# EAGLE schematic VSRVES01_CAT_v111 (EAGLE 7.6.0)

## Sheet 1 of 4: VSRV+DDR2
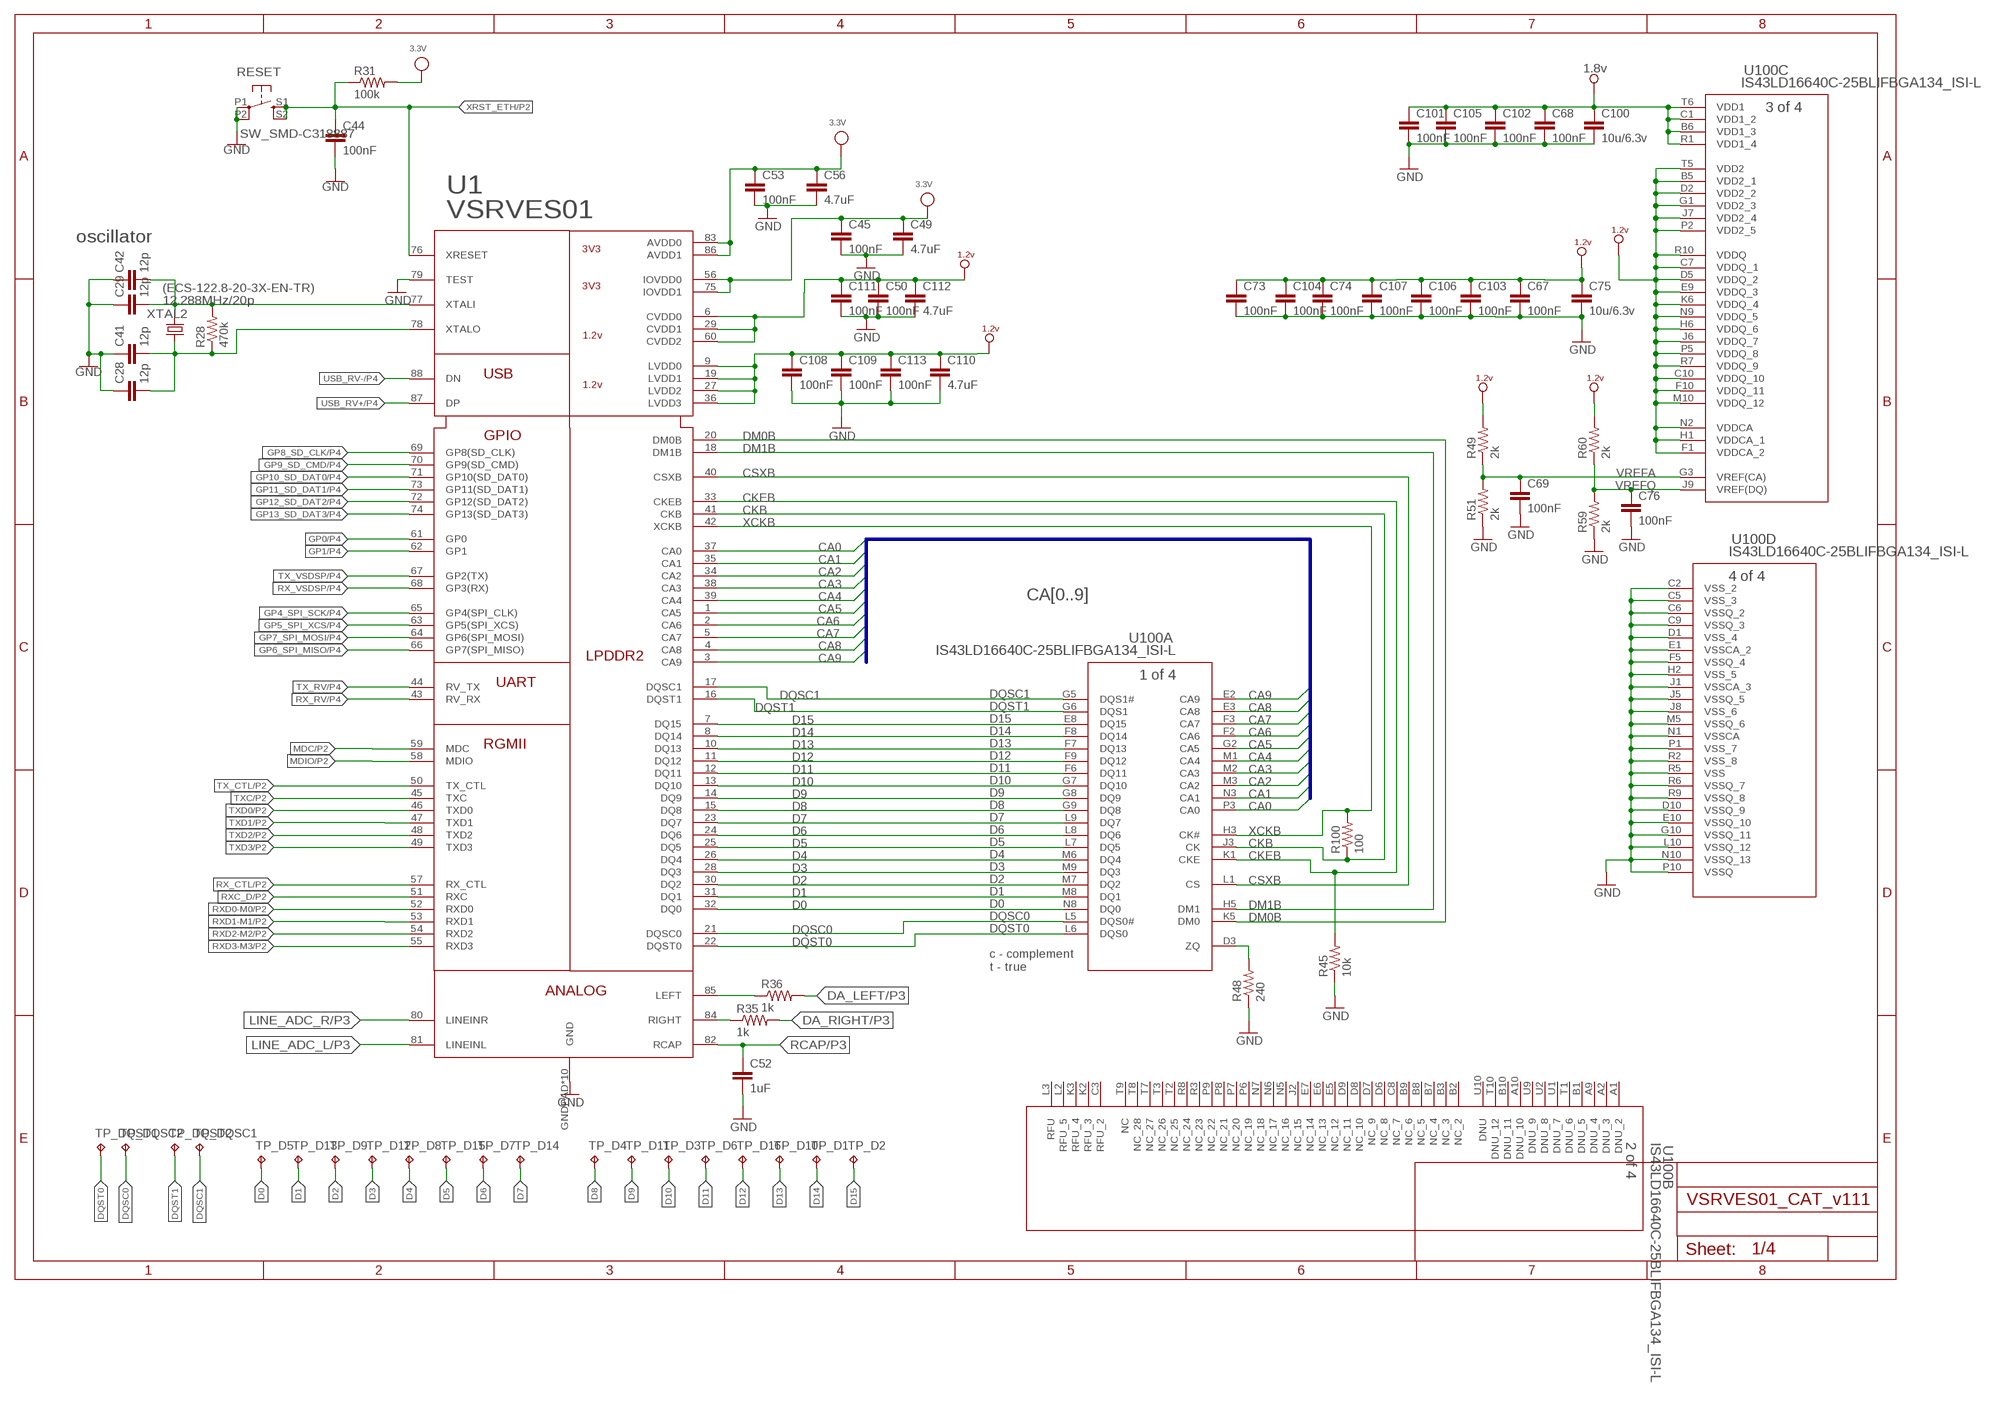
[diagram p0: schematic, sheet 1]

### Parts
C28  12p  C-EUC0603K  [C0603K]
C29  12p  C-EUC0603K  [C0603K]
C41  12p  C-EUC0603K  [C0603K]
C42  12p  C-EUC0603K  [C0603K]
C44  100nF  C-EUC0603K  [C0603K]
C45  100nF  C-EUC0603K  [C0603K]
C49  4.7uF  C-EUC0603K  [C0603K]
C50  100nF  C-EUC0603K  [C0603K]
C52  1uF  C-EUC0603K  [C0603K]
C53  100nF  C-EUC0603K  [C0603K]
C56  4.7uF  C-EUC0603K  [C0603K]
C67  100nF  C-EUC0603K  [C0603K]
C68  100nF  C-EUC0603K  [C0603K]
C69  100nF  C-EUC0603K  [C0603K]
C73  100nF  C-EUC0603K  [C0603K]
C74  100nF  C-EUC0603K  [C0603K]
C75  10u/6.3v  C-EUC0603K  [C0603K]
C76  100nF  C-EUC0603K  [C0603K]
C100  10u/6.3v  C-EUC0603K  [C0603K]
C101  100nF  C-EUC0603K  [C0603K]
C102  100nF  C-EUC0603K  [C0603K]
C103  100nF  C-EUC0603K  [C0603K]
C104  100nF  C-EUC0603K  [C0603K]
C105  100nF  C-EUC0603K  [C0603K]
C106  100nF  C-EUC0603K  [C0603K]
C107  100nF  C-EUC0603K  [C0603K]
C108  100nF  C-EUC0603K  [C0603K]
C109  100nF  C-EUC0603K  [C0603K]
C110  4.7uF  C-EUC0603K  [C0603K]
C111  100nF  C-EUC0603K  [C0603K]
C112  4.7uF  C-EUC0603K  [C0603K]
C113  100nF  C-EUC0603K  [C0603K]
R28  470k  R-US_R0603  [R0603]
R31  100k  R-US_R0603  [R0603]
R35  1k  R-US_R0603  [R0603]
R36  1k  R-US_R0603  [R0603]
R45  10k  R-US_R0603  [R0603]
R48  240  R-US_R0603  [R0603]
R49  2k  R-US_R0603  [R0603]
R51  2k  R-US_R0603  [R0603]
R59  2k  R-US_R0603  [R0603]
R60  2k  R-US_R0603  [R0603]
R100  100  R-US_R0603  [R0603]
RESET  SW_SMD-C318887  SW_SMD-SW-4_5.1X5.1X2.5_TS-1187A-C-E-B  [SW_SMD-SW-4_5.1X5.1X2.5_TS-1187A-C-E-B]
TP_D1  TPTP10R  [TP10R]
TP_D2  TPTP10R  [TP10R]
TP_D3  TPTP06R  [TP06R]
TP_D4  TPTP06R  [TP06R]
TP_D5  TPTP10R  [TP10R]
TP_D6  TPTP06R  [TP06R]
TP_D7  TPTP10R  [TP10R]
TP_D8  TPTP10R  [TP10R]
TP_D9  TPTP10R  [TP10R]
TP_D10  TPTP10R  [TP10R]
TP_D11  TPTP06R  [TP06R]
TP_D12  TPTP10R  [TP10R]
TP_D13  TPTP10R  [TP10R]
TP_D14  TPTP06R  [TP06R]
TP_D15  TPTP10R  [TP10R]
TP_D16  TPTP10R  [TP10R]
TP_DQSC1  TPTP06R  [TP06R]
TP_DQSC2  TPTP06R  [TP06R]
TP_DQST1  TPTP06R  [TP06R]
TP_DQST2  TPTP06R  [TP06R]
U1  VSRVES01  [QFN88_NEW2Q]
U100  IS43LD16640C-25BLIFBGA134_ISI-L  [FBGA134_ISI-L]
XTAL2  12.288MHz/20p  CRYSTAL  [CSM-3X]

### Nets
1.2V: C50.1 C67.1 C73.1 C74.1 C75.1 C103.1 C104.1 C106.1 C107.1 C108.1 C109.1 C110.1 C111.1 C112.1 C113.1 R49.2 R60.2 U1.6(CVDD0) U1.9(LVDD0) U1.19(LVDD1) U1.27(LVDD2) U1.29(CVDD1) U1.36(LVDD3) U1.60(CVDD2) U100.B5(C:VDD2_1) U100.C7(C:VDDQ_1) U100.C10(C:VDDQ_10) U100.D2(C:VDD2_2) U100.D5(C:VDDQ_2) U100.E9(C:VDDQ_3) U100.F1(C:VDDCA_2) U100.F10(C:VDDQ_11) U100.G1(C:VDD2_3) U100.H1(C:VDDCA_1) U100.H6(C:VDDQ_6) U100.J6(C:VDDQ_7) U100.J7(C:VDD2_4) U100.K6(C:VDDQ_4) U100.M10(C:VDDQ_12) U100.N2(C:VDDCA) U100.N9(C:VDDQ_5) U100.P2(C:VDD2_5) U100.P5(C:VDDQ_8) U100.R7(C:VDDQ_9) U100.R10(C:VDDQ) U100.T5(C:VDD2) ; supply symbol labelled +1.2V ; also sheet 2,4
1.8V: C68.1 C100.1 C101.1 C102.1 C105.1 U100.B6(C:VDD1_3) U100.C1(C:VDD1_2) U100.R1(C:VDD1_4) U100.T6(C:VDD1) ; supply symbol labelled +1.8V ; also sheet 4
3.3V: C45.1 C49.1 C53.1 C56.1 R31.2 U1.56(IOVDD0) U1.75(IOVDD1) U1.83(AVDD0) U1.86(AVDD1) ; also sheet 2,3,4
CA0: U1.37(CA0) U100.P3(A:CA0)
CA1: U1.35(CA1) U100.N3(A:CA1)
CA2: U1.34(CA2) U100.M3(A:CA2)
CA3: U1.38(CA3) U100.M2(A:CA3)
CA4: U1.39(CA4) U100.M1(A:CA4)
CA5: U1.1(CA5) U100.G2(A:CA5)
CA6: U1.2(CA6) U100.F2(A:CA6)
CA7: U1.5(CA7) U100.F3(A:CA7)
CA8: U1.4(CA8) U100.E3(A:CA8)
CA9: U1.3(CA9) U100.E2(A:CA9)
CKB: R100.1 U1.41(CKB) U100.J3(A:CK)
CKEB: R45.2 U1.33(CKEB) U100.K1(A:CKE)
CSXB: U1.40(CSXB) U100.L1(A:CS)
D0: TP_D5.TP U1.32(DQ0) U100.N8(A:DQ0)
D1: TP_D13.TP U1.31(DQ1) U100.M8(A:DQ1)
D2: TP_D9.TP U1.30(DQ2) U100.M7(A:DQ2)
D3: TP_D12.TP U1.28(DQ3) U100.M9(A:DQ3)
D4: TP_D8.TP U1.26(DQ4) U100.M6(A:DQ4)
D5: TP_D15.TP U1.25(DQ5) U100.L7(A:DQ5)
D6: TP_D7.TP U1.24(DQ6) U100.L8(A:DQ6)
D7: TP_D14.TP U1.23(DQ7) U100.L9(A:DQ7)
D8: TP_D4.TP U1.15(DQ8) U100.G9(A:DQ8)
D9: TP_D11.TP U1.14(DQ9) U100.G8(A:DQ9)
D10: TP_D3.TP U1.13(DQ10) U100.G7(A:DQ10)
D11: TP_D6.TP U1.12(DQ11) U100.F6(A:DQ11)
D12: TP_D16.TP U1.11(DQ12) U100.F9(A:DQ12)
D13: TP_D10.TP U1.10(DQ13) U100.F7(A:DQ13)
D14: TP_D1.TP U1.8(DQ14) U100.F8(A:DQ14)
D15: TP_D2.TP U1.7(DQ15) U100.E8(A:DQ15)
DA_LEFT: R36.2 ; also sheet 3
DA_RIGHT: R35.2 ; also sheet 3
DM0B: U1.20(DM0B) U100.K5(A:DM0)
DM1B: U1.18(DM1B) U100.H5(A:DM1)
DQSC0: TP_DQSC2.TP U1.21(DQSC0) U100.L5(A:DQS0#)
DQSC1: TP_DQSC1.TP U1.17(DQSC1) U100.G5(A:DQS1#)
DQST0: TP_DQST1.TP U1.22(DQST0) U100.L6(A:DQS0)
DQST1: TP_DQST2.TP U1.16(DQST1) U100.G6(A:DQS1)
GND: C28.1 C29.1 C41.1 C42.1 C44.2 C45.2 C49.2 C50.2 C52.2 C53.2 C56.2 C67.2 C68.2 C69.2 C73.2 C74.2 C75.2 C76.2 C100.2 C101.2 C102.2 C103.2 C104.2 C105.2 C106.2 C107.2 C108.2 C109.2 C110.2 C111.2 C112.2 C113.2 R45.1 R48.1 R51.1 R59.1 RESET.P1 RESET.P2 U1.79(TEST) U1.GNDPAD(GND) U1.P$1(GND) U1.P$2(GND) U1.P$3(GND) U1.P$4(GND) U1.P$5(GND) U1.P$6(GND) U1.P$7(GND) U1.P$8(GND) U1.P$9(GND) U100.C2(D:VSS_2) U100.C5(D:VSS_3) U100.C6(D:VSSQ_2) U100.C9(D:VSSQ_3) U100.D1(D:VSS_4) U100.D10(D:VSSQ_9) U100.E1(D:VSSCA_2) U100.E10(D:VSSQ_10) U100.F5(D:VSSQ_4) U100.G10(D:VSSQ_11) U100.H2(D:VSS_5) U100.J1(D:VSSCA_3) U100.J5(D:VSSQ_5) U100.J8(D:VSS_6) U100.L10(D:VSSQ_12) U100.M5(D:VSSQ_6) U100.N1(D:VSSCA) U100.N10(D:VSSQ_13) U100.P1(D:VSS_7) U100.P10(D:VSSQ) U100.R2(D:VSS_8) U100.R5(D:VSS) U100.R6(D:VSSQ_7) U100.R9(D:VSSQ_8) ; also sheet 2,3,4
GP0: U1.61(GP0) ; also sheet 4
GP1: U1.62(GP1) ; also sheet 4
GP4_SPI_SCK: U1.65(GP4(SPI_CLK)) ; also sheet 4
GP5_SPI_XCS: U1.63(GP5(SPI_XCS)) ; also sheet 4
GP6_SPI_MISO: U1.66(GP7(SPI_MISO)) ; also sheet 4
GP7_SPI_MOSI: U1.64(GP6(SPI_MOSI)) ; also sheet 4
GP8_SD_CLK: U1.69(GP8(SD_CLK)) ; also sheet 4
GP9_SD_CMD: U1.70(GP9(SD_CMD)) ; also sheet 4
GP10_SD_DAT0: U1.71(GP10(SD_DAT0)) ; also sheet 4
GP11_SD_DAT1: U1.73(GP11(SD_DAT1)) ; also sheet 4
GP12_SD_DAT2: U1.72(GP12(SD_DAT2)) ; also sheet 4
GP13_SD_DAT3: U1.74(GP13(SD_DAT3)) ; also sheet 4
LINE_ADC_L: U1.81(LINEINL) ; also sheet 3
LINE_ADC_R: U1.80(LINEINR) ; also sheet 3
MDC: U1.59(MDC) ; also sheet 2
MDIO: U1.58(MDIO) ; also sheet 2
N$202: R36.1 U1.85(LEFT)
N$203: R35.1 U1.84(RIGHT)
RCAP: C52.1 U1.82(RCAP) ; also sheet 3
RX_CTL: U1.57(RX_CTL) ; also sheet 2
RX_RV: U1.43(RV_RX) ; also sheet 4
RX_VSDSP: U1.68(GP3(RX)) ; also sheet 4
RXC_D: U1.51(RXC) ; also sheet 2
RXD0-M0: U1.52(RXD0) ; also sheet 2
RXD1-M1: U1.53(RXD1) ; also sheet 2
RXD2-M2: U1.54(RXD2) ; also sheet 2
RXD3-M3: U1.55(RXD3) ; also sheet 2
TX_CTL: U1.50(TX_CTL) ; also sheet 2
TX_RV: U1.44(RV_TX) ; also sheet 4
TX_VSDSP: U1.67(GP2(TX)) ; also sheet 4
TXC: U1.45(TXC) ; also sheet 2
TXD0: U1.46(TXD0) ; also sheet 2
TXD1: U1.47(TXD1) ; also sheet 2
TXD2: U1.48(TXD2) ; also sheet 2
TXD3: U1.49(TXD3) ; also sheet 2
USB_RV+: U1.87(DP) ; also sheet 4
USB_RV-: U1.88(DN) ; also sheet 4
VREFA: C69.1 R49.1 R51.2 U100.G3(C:VREF(CA))
VREFQ: C76.1 R59.2 R60.1 U100.J9(C:VREF(DQ))
XCKB: R100.2 U1.42(XCKB) U100.H3(A:CK#)
XRST_ETH: C44.1 R31.1 RESET.S1 RESET.S2 U1.76(XRESET) ; also sheet 2
XTALI_UI: C29.2 C42.2 R28.2 U1.77(XTALI) XTAL2.2
XTALO_UI: C28.2 C41.2 R28.1 U1.78(XTALO) XTAL2.1
ZQ1: R48.2 U100.D3(A:ZQ)
Unconnected: U100.A1(B:DNU_2) U100.A2(B:DNU_3) U100.A9(B:DNU_4) U100.A10(B:DNU_10) U100.B1(B:DNU_5) U100.B2(B:NC_2) U100.B3(B:NC_3) U100.B7(B:NC_4) U100.B8(B:NC_5) U100.B9(B:NC_6) U100.B10(B:DNU_11) U100.C3(B:RFU_2) U100.C8(B:NC_7) U100.D6(B:NC_8) U100.D7(B:NC_9) U100.D8(B:NC_10) U100.D9(B:NC_11) U100.E5(B:NC_12) U100.E6(B:NC_13) U100.E7(B:NC_14) U100.J2(B:NC_15) U100.K2(B:RFU_3) U100.K3(B:RFU_4) U100.L2(B:RFU_5) U100.L3(B:RFU) U100.N5(B:NC_16) U100.N6(B:NC_17) U100.N7(B:NC_18) U100.P6(B:NC_19) U100.P7(B:NC_20) U100.P8(B:NC_21) U100.P9(B:NC_22) U100.R3(B:NC_23) U100.R8(B:NC_24) U100.T1(B:DNU_6) U100.T2(B:NC_25) U100.T3(B:NC_26) U100.T7(B:NC_27) U100.T8(B:NC_28) U100.T9(B:NC) U100.T10(B:DNU_12) U100.U1(B:DNU_7) U100.U2(B:DNU_8) U100.U9(B:DNU_9) U100.U10(B:DNU)

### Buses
CA[0..9]

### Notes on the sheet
- oscillator
- (ECS-122.8-20-3X-EN-TR)
- c - complement
  t - true

## Sheet 2 of 4: RGMII
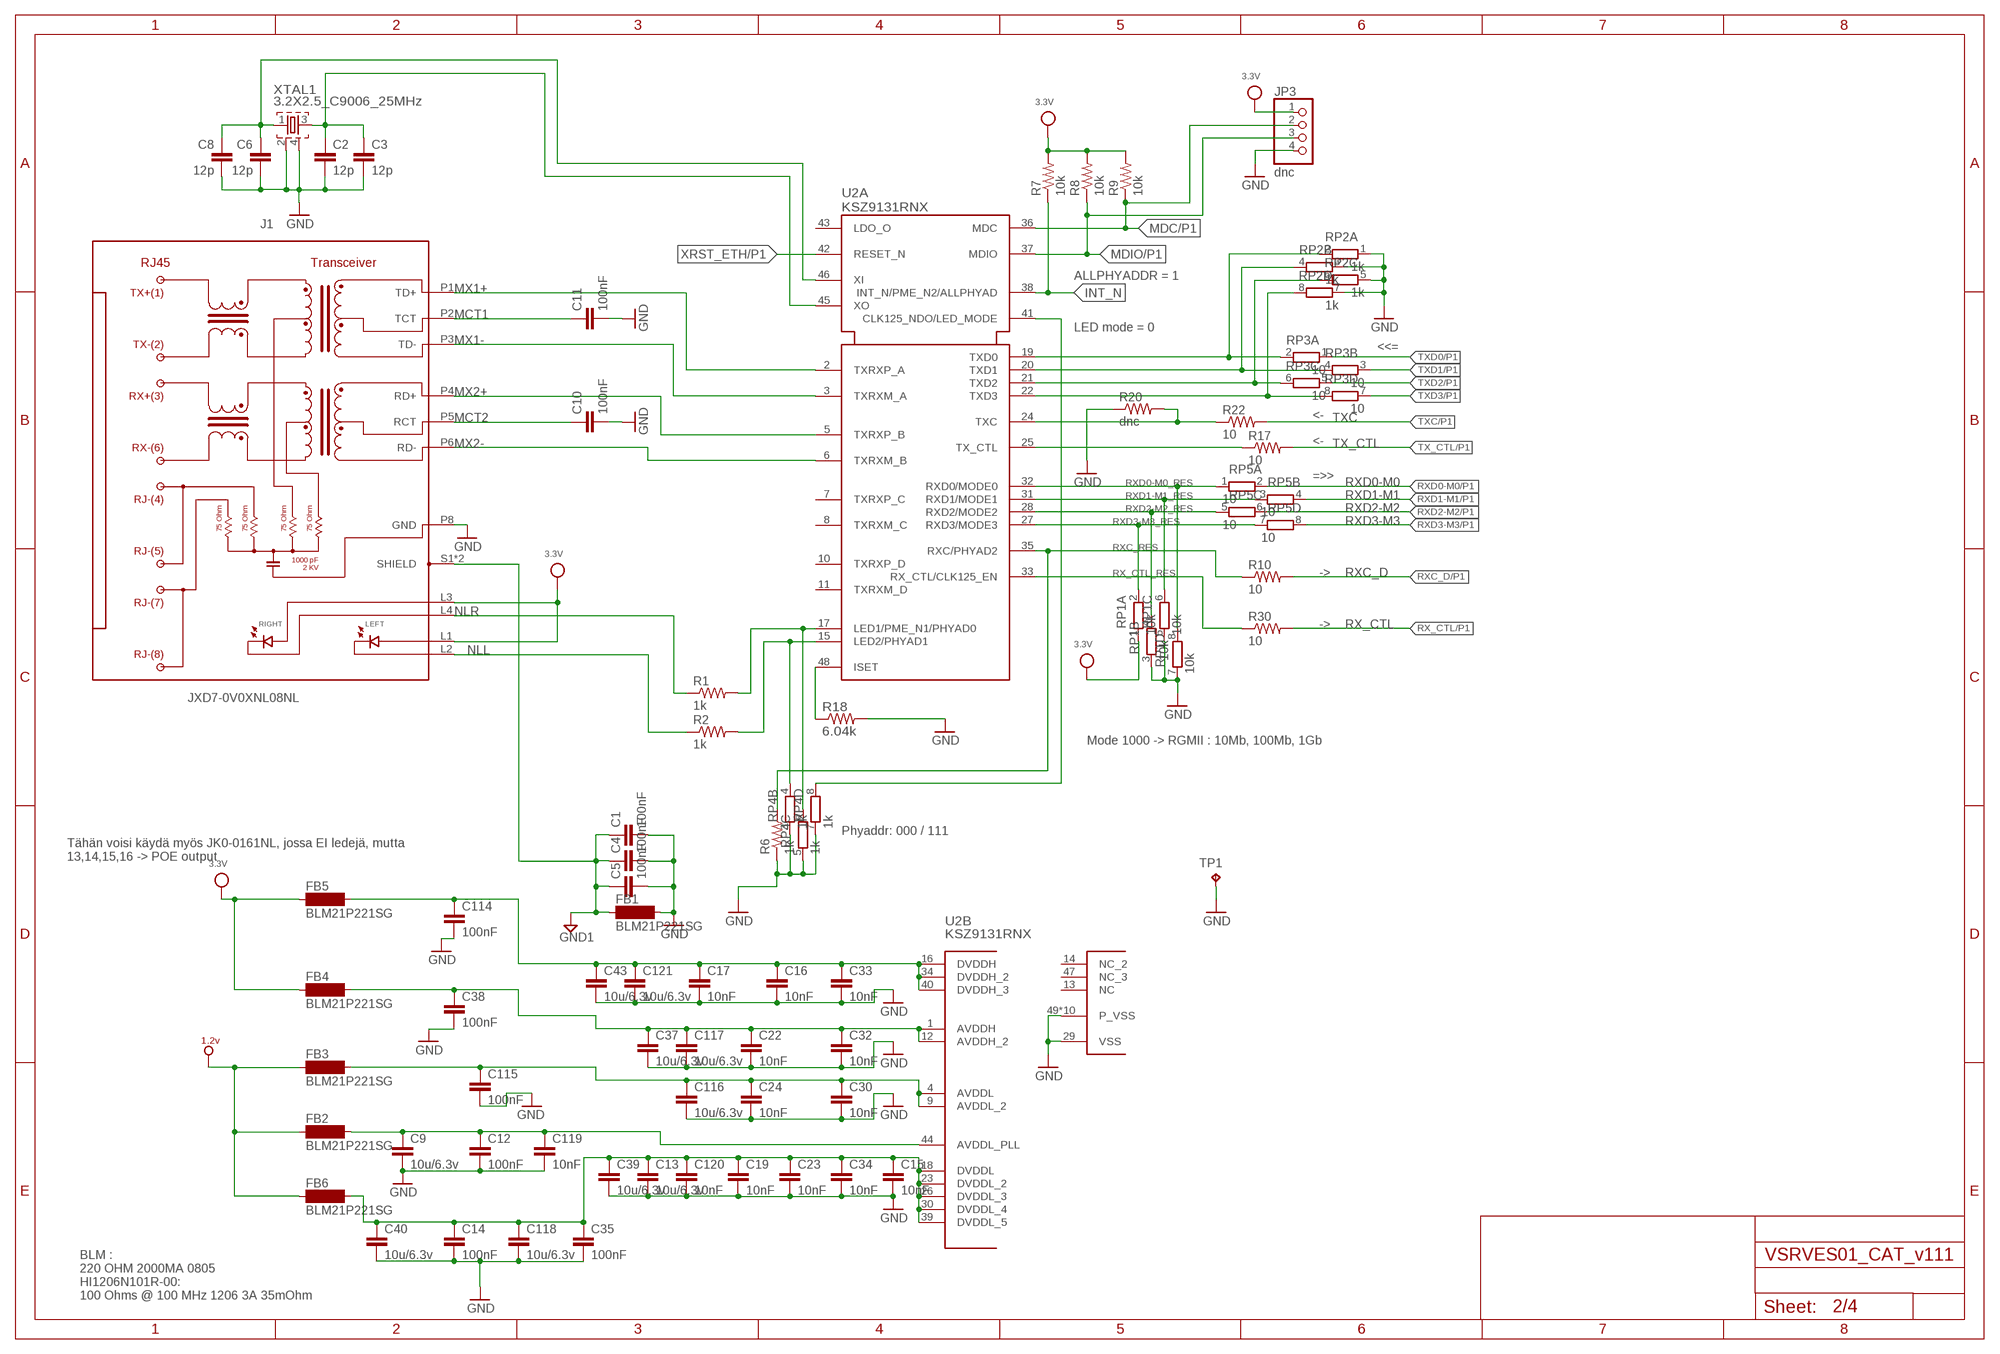
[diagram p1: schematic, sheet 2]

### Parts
C1  100nF  C-EUC0603K  [C0603K]
C2  12p  C-EUC0603K  [C0603K]
C3  12p  C-EUC0603K  [C0603K]
C4  100nF  C-EUC0603K  [C0603K]
C5  100nF  C-EUC0603K  [C0603K]
C6  12p  C-EUC0603K  [C0603K]
C8  12p  C-EUC0603K  [C0603K]
C9  10u/6.3v  C-EUC0603K  [C0603K]
C10  100nF  C-EUC0603K  [C0603K]
C11  100nF  C-EUC0603K  [C0603K]
C12  100nF  C-EUC0603K  [C0603K]
C13  10u/6.3v  C-EUC0603K  [C0603K]
C14  100nF  C-EUC0603K  [C0603K]
C15  10nF  C-EUC0603K  [C0603K]
C16  10nF  C-EUC0603K  [C0603K]
C17  10nF  C-EUC0603K  [C0603K]
C19  10nF  C-EUC0603K  [C0603K]
C22  10nF  C-EUC0603K  [C0603K]
C23  10nF  C-EUC0603K  [C0603K]
C24  10nF  C-EUC0603K  [C0603K]
C30  10nF  C-EUC0603K  [C0603K]
C32  10nF  C-EUC0603K  [C0603K]
C33  10nF  C-EUC0603K  [C0603K]
C34  10nF  C-EUC0603K  [C0603K]
C35  100nF  C-EUC0603K  [C0603K]
C37  10u/6.3v  C-EUC0603K  [C0603K]
C38  100nF  C-EUC0603K  [C0603K]
C39  10u/6.3v  C-EUC0603K  [C0603K]
C40  10u/6.3v  C-EUC0603K  [C0603K]
C43  10u/6.3v  C-EUC0603K  [C0603K]
C114  100nF  C-EUC0603K  [C0603K]
C115  100nF  C-EUC0603K  [C0603K]
C116  10u/6.3v  C-EUC0603K  [C0603K]
C117  10u/6.3v  C-EUC0603K  [C0603K]
C118  10u/6.3v  C-EUC0603K  [C0603K]
C119  10nF  C-EUC0603K  [C0603K]
C120  10nF  C-EUC0603K  [C0603K]
C121  10u/6.3v  C-EUC0603K  [C0603K]
FB1  BLM21P221SG  BLM  [L0805]
FB2  BLM21P221SG  BLM  [L0805]
FB3  BLM21P221SG  BLM  [L0805]
FB4  BLM21P221SG  BLM  [L0805]
FB5  BLM21P221SG  BLM  [L0805]
FB6  BLM21P221SG  BLM  [L0805]
J1  JXD7-0V0XNL08NL  [JXD7]
JP3  dnc  PINHD-1X4  [1X04]
R1  1k  R-US_R0603  [R0603]
R2  1k  R-US_R0603  [R0603]
R6  1k  R-US_R0603  [R0603]
R7  10k  R-US_R0603  [R0603]
R8  10k  R-US_R0603  [R0603]
R9  10k  R-US_R0603  [R0603]
R10  10  R-US_R0603  [R0603]
R17  10  R-US_R0603  [R0603]
R18  6.04k  R-US_R1206  [R1206]
R20  dnc  R-US_R0603  [R0603]
R22  10  R-US_R0603  [R0603]
R30  10  R-US_R0603  [R0603]
RP1  10k  RESPAK-4X1206  [RAS_ARR_1206]
RP2  1k  RESPAK-4X1206  [RAS_ARR_1206]
RP3  10  RESPAK-4X1206  [RAS_ARR_1206]
RP4  1k  RESPAK-4X1206  [RAS_ARR_1206]
RP5  10  RESPAK-4X1206  [RAS_ARR_1206]
TP1  TPPAD1-13  [P1-13]
U2  KSZ9131RNX  [48-VFQFN_7X7]
XTAL1  3.2X2.5_C9006_25MHz  CRYSTAL_3.2X2.5_NEW  [3.2X2.5_CRYSTAL]

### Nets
1.2V: FB2.1 FB3.1 FB6.1 ; supply symbol labelled +1.2V ; also sheet 1,4
3.3V: FB4.1 FB5.1 J1.L1 J1.L3 JP3.1 R7.2 R8.2 R9.2 RP1.1 ; also sheet 1,3,4
GND: C1.2 C2.2 C3.2 C4.2 C5.2 C6.2 C8.2 C9.2 C10.2 C11.2 C12.2 C13.2 C14.2 C15.2 C16.2 C17.2 C19.2 C22.2 C23.2 C24.2 C30.2 C32.2 C33.2 C34.2 C35.2 C37.2 C38.2 C39.2 C40.2 C43.2 C114.2 C115.2 C116.2 C117.2 C118.2 C119.2 C120.2 C121.2 FB1.2 J1.P8(GND) JP3.4 R6.1 R18.2 R20.1 RP1.3 RP1.5 RP1.7 RP2.1 RP2.3 RP2.5 RP2.7 RP4.3 RP4.5 RP4.7 TP1.TP U2.29(B:VSS) U2.49(B:P_VSS) U2.G1(B:P_VSS) U2.G2(B:P_VSS) U2.G3(B:P_VSS) U2.G4(B:P_VSS) U2.G5(B:P_VSS) U2.G6(B:P_VSS) U2.G7(B:P_VSS) U2.G8(B:P_VSS) U2.G9(B:P_VSS) XTAL1.2 XTAL1.4 ; also sheet 1,3,4
GND1: C1.1 C4.1 C5.1 FB1.1 J1.S1(SHIELD) J1.S2(SHIELD)
INT_N: R7.1 U2.38(A:INT_N/PME_N2/ALLPHYAD)
MCT1: C11.1 J1.P2(TCT)
MCT2: C10.1 J1.P5(RCT)
MDC: JP3.2 R9.1 U2.36(A:MDC) ; also sheet 1
MDIO: JP3.3 R8.1 U2.37(A:MDIO) ; also sheet 1
MX1+: J1.P1(TD+) U2.2(A:TXRXP_A)
MX1-: J1.P3(TD-) U2.3(A:TXRXM_A)
MX2+: J1.P4(RD+) U2.5(A:TXRXP_B)
MX2-: J1.P6(RD-) U2.6(A:TXRXM_B)
N$2: C16.1 C17.1 C33.1 C43.1 C114.1 C121.1 FB5.2 U2.16(B:DVDDH) U2.34(B:DVDDH_2) U2.40(B:DVDDH_3)
N$5: C22.1 C32.1 C37.1 C38.1 C117.1 FB4.2 U2.1(B:AVDDH) U2.12(B:AVDDH_2)
N$8: C24.1 C30.1 C115.1 C116.1 FB3.2 U2.4(B:AVDDL) U2.9(B:AVDDL_2)
N$9: C9.1 C12.1 C119.1 FB2.2 U2.44(B:AVDDL_PLL)
N$15: C13.1 C14.1 C15.1 C19.1 C23.1 C34.1 C35.1 C39.1 C40.1 C118.1 C120.1 FB6.2 U2.18(B:DVDDL) U2.23(B:DVDDL_2) U2.26(B:DVDDL_3) U2.30(B:DVDDL_4) U2.39(B:DVDDL_5)
N$75: R1.2 RP4.6 U2.17(A:LED1/PME_N1/PHYAD0)
N$77: R2.2 RP4.4 U2.15(A:LED2/PHYAD1)
N$78: RP2.2 RP3.2 U2.19(A:TXD0)
N$79: RP2.4 RP3.4 U2.20(A:TXD1)
N$80: RP2.6 RP3.6 U2.21(A:TXD2)
N$81: RP2.8 RP3.8 U2.22(A:TXD3)
N$82: R20.2 R22.1 U2.24(A:TXC)
N$83: R17.1 U2.25(A:TX_CTL)
N$93: RP4.8 U2.41(A:CLK125_NDO/LED_MODE)
N$95: R18.1 U2.48(A:ISET)
NLL: J1.L2 R2.1
NLR: J1.L4 R1.1
Q1N1: C2.1 C3.1 U2.45(A:XO) XTAL1.3
Q1P1: C6.1 C8.1 U2.46(A:XI) XTAL1.1
RX_CTL: R30.2 ; also sheet 1
RX_CTL_RES: R30.1 U2.33(A:RX_CTL/CLK125_EN)
RXC_D: R10.2 ; also sheet 1
RXC_RES: R6.2 R10.1 U2.35(A:RXC/PHYAD2)
RXD0-M0: RP5.2 ; also sheet 1
RXD0-M0_RES: RP1.8 RP5.1 U2.32(A:RXD0/MODE0)
RXD1-M1: RP5.4 ; also sheet 1
RXD1-M1_RES: RP1.6 RP5.3 U2.31(A:RXD1/MODE1)
RXD2-M2: RP5.6 ; also sheet 1
RXD2-M2_RES: RP1.4 RP5.5 U2.28(A:RXD2/MODE2)
RXD3-M3: RP5.8 ; also sheet 1
RXD3-M3_RES: RP1.2 RP5.7 U2.27(A:RXD3/MODE3)
TX_CTL: R17.2 ; also sheet 1
TXC: R22.2 ; also sheet 1
TXD0: RP3.1 ; also sheet 1
TXD1: RP3.3 ; also sheet 1
TXD2: RP3.5 ; also sheet 1
TXD3: RP3.7 ; also sheet 1
XRST_ETH: U2.42(A:RESET_N) ; also sheet 1
Unconnected: RP4.1 RP4.2 U2.7(A:TXRXP_C) U2.8(A:TXRXM_C) U2.10(A:TXRXP_D) U2.11(A:TXRXM_D) U2.13(B:NC) U2.14(B:NC_2) U2.43(A:LDO_O) U2.47(B:NC_3)

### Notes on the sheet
- ALLPHYADDR = 1
- LED mode = 0
- <<=
- <-
- <-
- =>>
- ->
- ->
- Mode 1000 -> RGMII : 10Mb, 100Mb, 1Gb
- Phyaddr: 000 / 111
- Tähän voisi käydä myös JK0-0161NL, jossa EI ledejä, mutta
  13,14,15,16 -> POE output
- BLM :
  220 OHM 2000MA 0805
  HI1206N101R-00: 
  100 Ohms @ 100 MHz 1206 3A 35mOhm

## Sheet 3 of 4: analog
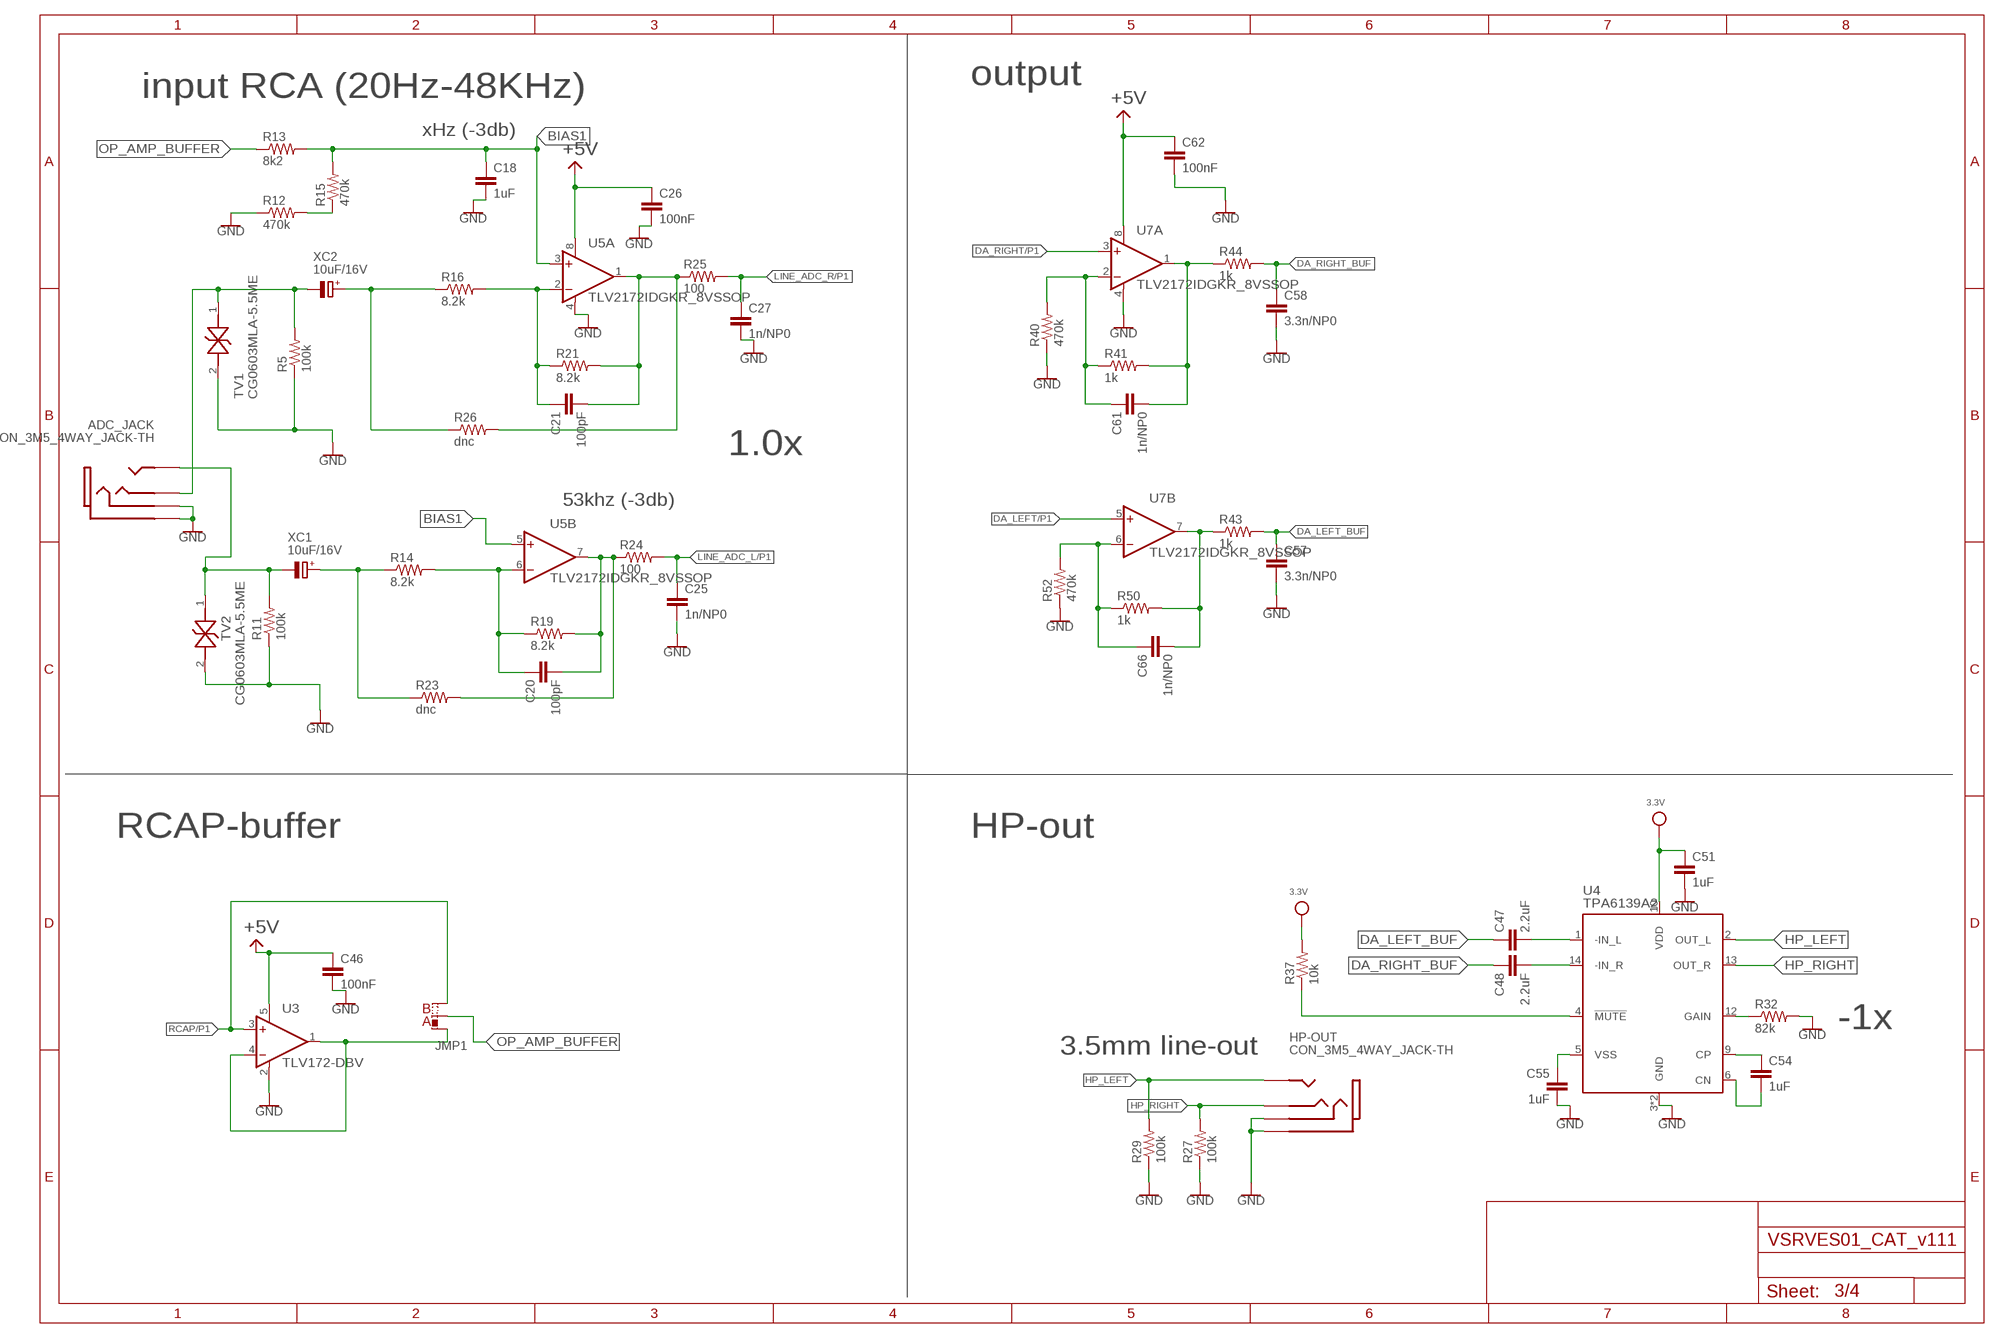
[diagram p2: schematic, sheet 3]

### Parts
ADC_JACK  CON_3M5_4WAY_JACK-TH  [SJ-43514B]
C18  1uF  C-EUC0603K  [C0603K]
C20  100pF  C-EUC0603K  [C0603K]
C21  100pF  C-EUC0603K  [C0603K]
C25  1n/NP0  C-EUC0603K  [C0603K]
C26  100nF  C-EUC0603K  [C0603K]
C27  1n/NP0  C-EUC0603K  [C0603K]
C46  100nF  C-EUC0603K  [C0603K]
C47  2.2uF  C-EUC0603K  [C0603K]
C48  2.2uF  C-EUC0603K  [C0603K]
C51  1uF  C-EUC0603K  [C0603K]
C54  1uF  C-EUC0603K  [C0603K]
C55  1uF  C-EUC0603K  [C0603K]
C57  3.3n/NP0  C-EUC0603K  [C0603K]
C58  3.3n/NP0  C-EUC0603K  [C0603K]
C61  1n/NP0  C-EUC0603K  [C0603K]
C62  100nF  C-EUC0603K  [C0603K]
C66  1n/NP0  C-EUC0603K  [C0603K]
HP-OUT  CON_3M5_4WAY_JACK-TH  [SJ-43514B]
JMP1  0R-JMPR  [0603X2]
R5  100k  R-US_R0603  [R0603]
R11  100k  R-US_R0603  [R0603]
R12  470k  R-US_R0603  [R0603]
R13  8k2  R-US_R0603  [R0603]
R14  8.2k  R-US_R0603  [R0603]
R15  470k  R-US_R0603  [R0603]
R16  8.2k  R-US_R0603  [R0603]
R19  8.2k  R-US_R0603  [R0603]
R21  8.2k  R-US_R0603  [R0603]
R23  dnc  R-US_R0603  [R0603]
R24  100  R-US_R0603  [R0603]
R25  100  R-US_R0603  [R0603]
R26  dnc  R-US_R0603  [R0603]
R27  100k  R-US_R0603  [R0603]
R29  100k  R-US_R0603  [R0603]
R32  82k  R-US_R0603  [R0603]
R37  10k  R-US_R0603  [R0603]
R40  470k  R-US_R0603  [R0603]
R41  1k  R-US_R0603  [R0603]
R43  1k  R-US_R0603  [R0603]
R44  1k  R-US_R0603  [R0603]
R50  1k  R-US_R0603  [R0603]
R52  470k  R-US_R0603  [R0603]
TV1  CG0603MLA-5.5ME  [0603]
TV2  CG0603MLA-5.5ME  [0603]
U3  TLV172-DBV  [SOT23-5]
U4  TPA6139A2  [TSSOP-14_4.4MM]
U5  TLV2172IDGKR_8VSSOP  [8-VSSOP]
U7  TLV2172IDGKR_8VSSOP  [8-VSSOP]
XC1  10uF/16V  CPOL-EUB  [EC-SMD-44X44]
XC2  10uF/16V  CPOL-EUB  [EC-SMD-44X44]

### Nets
3.3V: C51.1 R37.2 U4.10(VDD) ; also sheet 1,2,4
+5V: C26.1 C46.1 C62.1 U3.5(V+) U5.8(A:V+) U7.8(A:V+) ; also sheet 4
BIAS1: C18.1 R13.2 R15.2 U5.3(A:+IN) U5.5(B:+IN)
DA_LEFT: U7.5(B:+IN) ; also sheet 1
DA_LEFT_BUF: C47.1 C57.1 R43.2
DA_RIGHT: U7.3(A:+IN) ; also sheet 1
DA_RIGHT_BUF: C48.1 C58.1 R44.2
GND: ADC_JACK.5(GND) ADC_JACK.6(POLE4) C18.2 C25.2 C26.2 C27.2 C46.2 C51.2 C55.2 C57.2 C58.2 C62.2 HP-OUT.5(GND) HP-OUT.6(POLE4) R5.1 R11.1 R12.1 R27.1 R29.1 R32.2 R40.1 R52.1 TV1.2(A2) TV2.2(A2) U3.2(V-) U4.3(GND) U4.11(GND) U5.4(A:V-) U7.4(A:V-) ; also sheet 1,2,4
HP_LEFT: HP-OUT.4(LEFT) R29.2 U4.2(OUT_L)
HP_MUTE: R37.1 U4.4(!MUTE)
HP_RIGHT: HP-OUT.1(RIGHT) R27.2 U4.13(OUT_R)
LINE_ADC_L: C25.1 R24.2 ; also sheet 1
LINE_ADC_R: C27.1 R25.2 ; also sheet 1
N$1: JMP1.1 U3.1(OUT) U3.4(-IN)
N$3: C66.2 R43.1 R50.2 U7.7(B:OUT)
N$4: C61.2 R41.2 R44.1 U7.1(A:OUT)
N$11: C21.1 R16.2 R21.1 U5.2(A:-IN)
N$12: R16.1 R26.1 XC2.+
N$13: R14.1 R23.1 XC1.+
N$14: ADC_JACK.4(LEFT) R11.2 TV2.1(A1) XC1.-
N$18: R12.2 R15.1
N$20: ADC_JACK.1(RIGHT) R5.2 TV1.1(A1) XC2.-
N$27: C61.1 R40.2 R41.1 U7.2(A:-IN)
N$30: C66.1 R50.1 R52.2 U7.6(B:-IN)
N$45: C20.2 R19.2 R23.2 R24.1 U5.7(B:OUT)
N$46: C21.2 R21.2 R25.1 R26.2 U5.1(A:OUT)
N$48: C20.1 R14.2 R19.1 U5.6(B:-IN)
N$178: C55.1 U4.5(VSS)
N$181: C48.2 U4.14(-IN_R)
N$182: C47.2 U4.1(-IN_L)
N$185: R32.1 U4.12(GAIN)
N$186: C54.1 U4.9(CP)
N$187: C54.2 U4.6(CN)
OP_AMP_BUFFER: JMP1.2 R13.1
RCAP: JMP1.3 U3.3(+IN) ; also sheet 1

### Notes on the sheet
- output
- input RCA (20Hz-48KHz)
- xHz (-3db)
- 1.0x
- 53khz (-3db)
- RCAP-buffer | HP-out
- -1x
- 3.5mm line-out

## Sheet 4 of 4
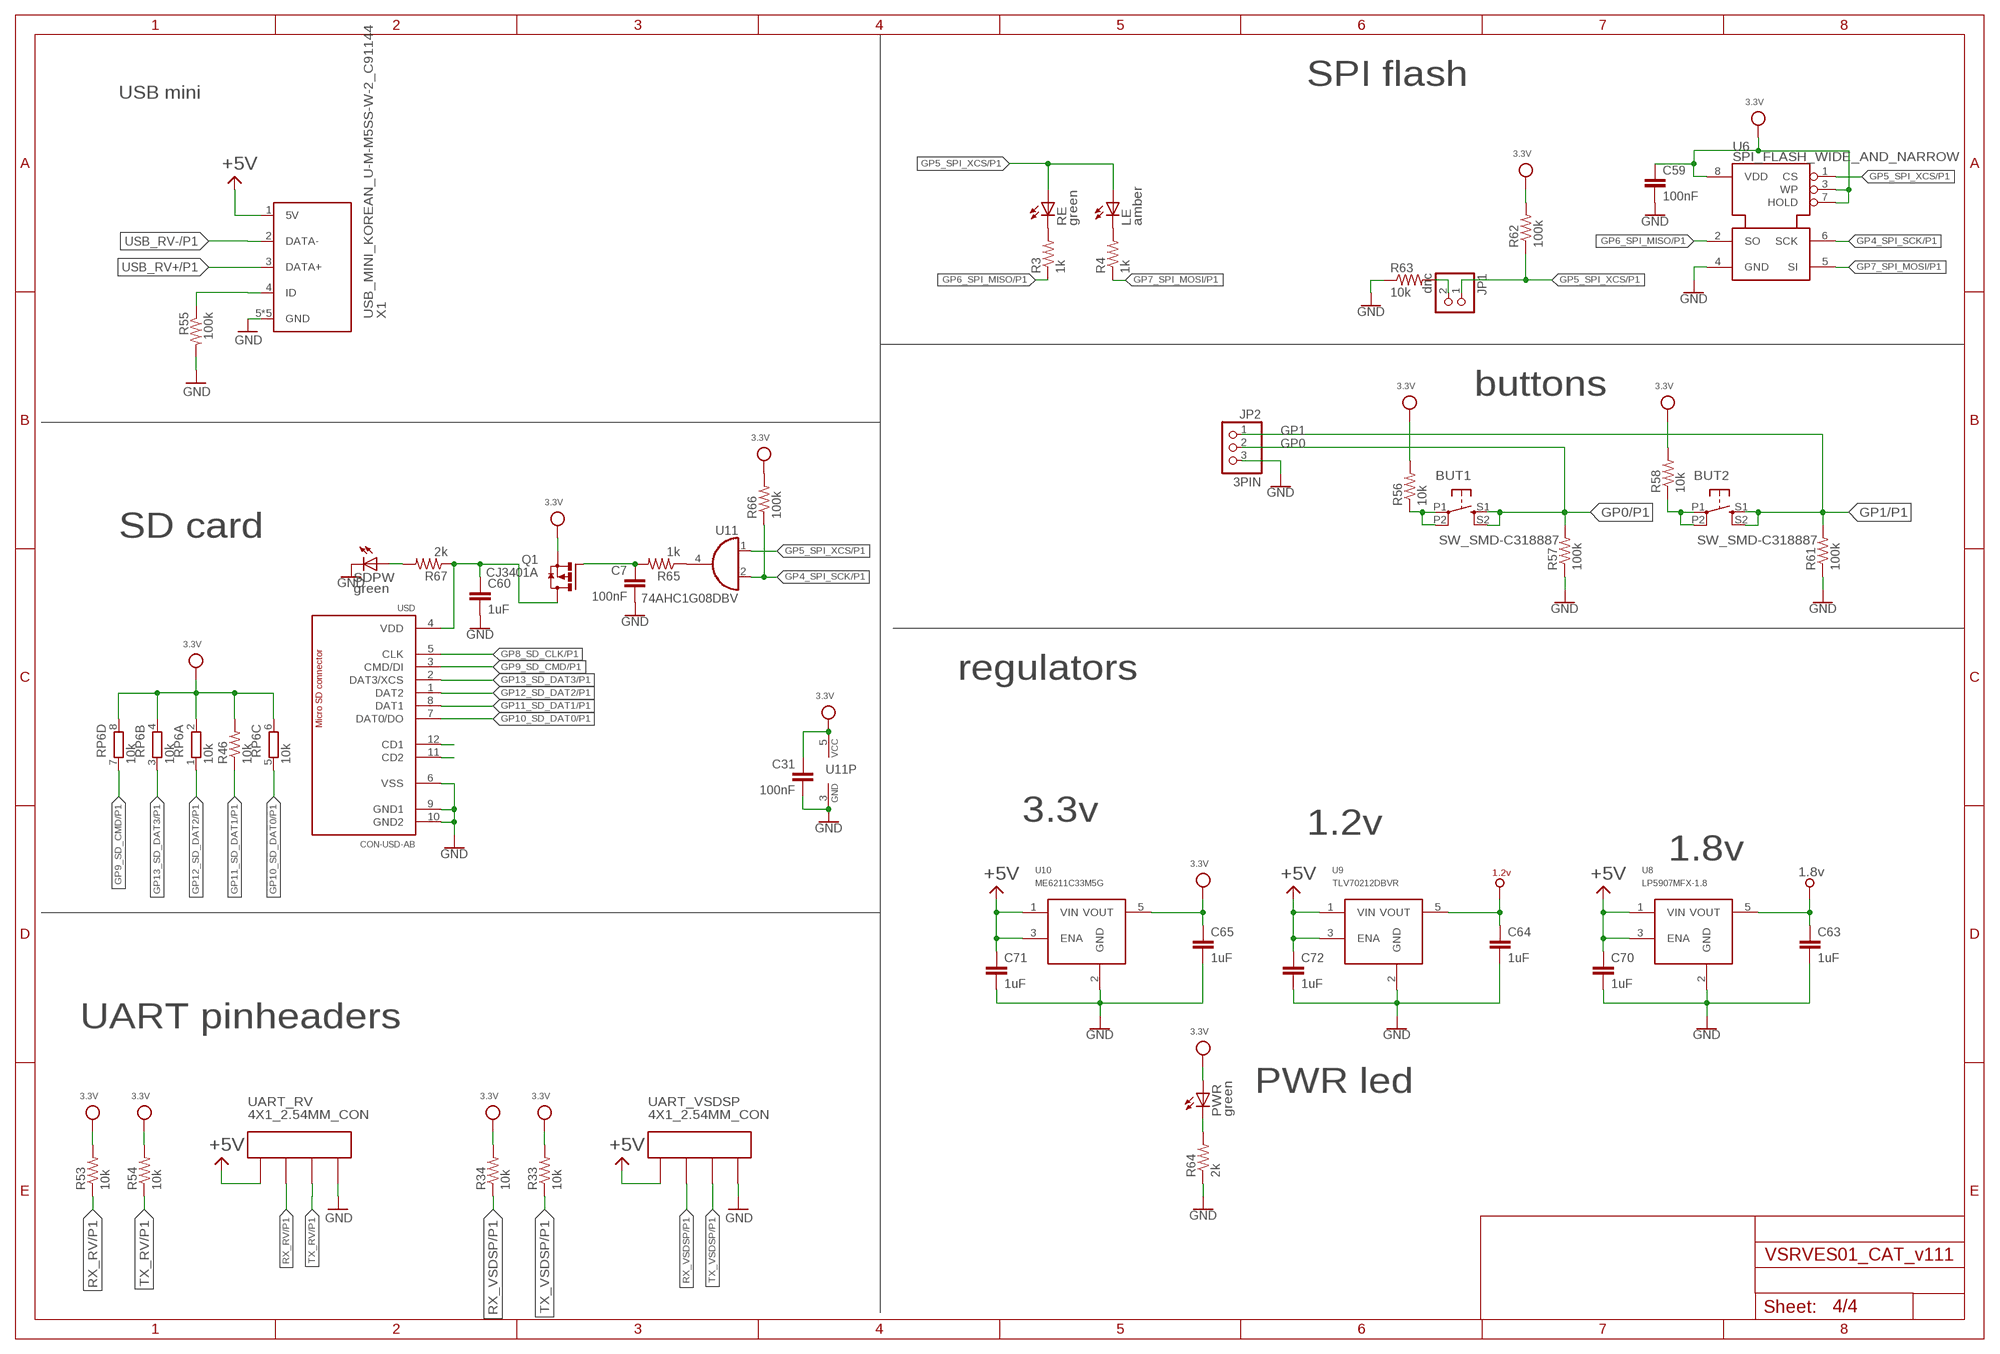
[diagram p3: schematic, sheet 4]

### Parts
BUT1  SW_SMD-C318887  SW_SMD-SW-4_5.1X5.1X2.5_TS-1187A-C-E-B  [SW_SMD-SW-4_5.1X5.1X2.5_TS-1187A-C-E-B]
BUT2  SW_SMD-C318887  SW_SMD-SW-4_5.1X5.1X2.5_TS-1187A-C-E-B  [SW_SMD-SW-4_5.1X5.1X2.5_TS-1187A-C-E-B]
C7  100nF  C-EUC0603K  [C0603K]
C31  100nF  C-EUC0603K  [C0603K]
C59  100nF  C-EUC0603K  [C0603K]
C60  1uF  C-EUC0603  [C0603]
C63  1uF  C-EUC0603K  [C0603K]
C64  1uF  C-EUC0603K  [C0603K]
C65  1uF  C-EUC0603K  [C0603K]
C70  1uF  C-EUC0603K  [C0603K]
C71  1uF  C-EUC0603K  [C0603K]
C72  1uF  C-EUC0603K  [C0603K]
JP1  dnc  PINHD-1X2  [1X02]
JP2  3PIN  PINHD-1X3  [1X03]
LE  amber  LED_0603  [LED_0603]
PWR  green  LED_0603  [LED_0603]
Q1  CJ3401A  DMP3098L  [SOT23]
R3  1k  R-US_R0603  [R0603]
R4  1k  R-US_R0603  [R0603]
R33  10k  R-US_R0603  [R0603]
R34  10k  R-US_R0603  [R0603]
R46  10k  R-US_R0603  [R0603]
R53  10k  R-US_R0603  [R0603]
R54  10k  R-US_R0603  [R0603]
R55  100k  R-US_R0603  [R0603]
R56  10k  R-US_R0603  [R0603]
R57  100k  R-US_R0603  [R0603]
R58  10k  R-US_R0603  [R0603]
R61  100k  R-US_R0603  [R0603]
R62  100k  R-US_R0603  [R0603]
R63  10k  R-US_R0603  [R0603]
R64  2k  R-US_R0603  [R0603]
R65  1k  R-US_R0603  [R0603]
R66  100k  R-US_R0603  [R0603]
R67  2k  R-US_R0603  [R0603]
RE  green  LED_0603  [LED_0603]
RP6  10k  RESPAK-4X1206  [RAS_ARR_1206]
SDPW  green  LED_0603  [LED_0603]
U6  SPI_FLASH_WIDE_AND_NARROW  [SO-08M_WIDE]
U8  LP5907MFX-1.8  ZXCL280E5TA  [SOT23-5L]
U9  TLV70212DBVR  ZXCL280E5TA  [SOT23-5L]
U10  ME6211C33M5G  ZXCL280E5TA  [SOT23-5L]
U11  74AHC1G08DBV  [SOT23-5]
UART_RV  4X1_2.54MM_CON  [4X1_2.54MM_CON]
UART_VSDSP  4X1_2.54MM_CON  [4X1_2.54MM_CON]
USD  CON-USD-AB  [47(309/571)]
X1  USB_MINI_KOREAN_U-M-M5SS-W-2_C91144  [MINI_USB_KOREAN_HROPARTS_U-M-M5SS-W-2_C91144]

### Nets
1.2V: C64.1 U9.5(VOUT) ; supply symbol labelled +1.2V ; also sheet 1,2
1.8V: C63.1 U8.5(VOUT) ; supply symbol labelled +1.8V ; also sheet 1
3.3V: C31.1 C59.1 C65.1 PWR.A Q1.2(S) R33.2 R34.2 R46.2 R53.2 R54.2 R56.2 R58.2 R62.2 R66.2 RP6.2 RP6.4 RP6.6 RP6.8 U6.3(WP) U6.7(HOLD) U6.8(VDD) U10.5(VOUT) U11.5(VCC) ; also sheet 1,2,3
+5V: C70.1 C71.1 C72.1 U8.1(VIN) U8.3(ENA) U9.1(VIN) U9.3(ENA) U10.1(VIN) U10.3(ENA) UART_RV.P$1 UART_VSDSP.P$1 X1.1(5V) ; also sheet 3
GND: C7.2 C31.2 C59.2 C60.2 C63.2 C64.2 C65.2 C70.2 C71.2 C72.2 JP2.3 R55.2 R57.1 R61.1 R63.1 R64.1 SDPW.C U6.4(GND) U8.2(GND) U9.2(GND) U10.2(GND) U11.3(GND) UART_RV.P$4 UART_VSDSP.P$4 USD.6(VSS) USD.9(GND1) USD.10(GND2) X1.5(GND) X1.G1(GND) X1.G2(GND) X1.G3(GND) X1.G4(GND) ; also sheet 1,2,3
GP0: BUT1.S1 BUT1.S2 JP2.2 R57.2 ; also sheet 1
GP1: BUT2.S1 BUT2.S2 JP2.1 R61.2 ; also sheet 1
GP4_SPI_SCK: R66.1 U6.6(SCK) U11.2(I1) ; also sheet 1
GP5_SPI_XCS: JP1.1 LE.A R62.1 RE.A U6.1(CS) U11.1(I0) ; also sheet 1
GP6_SPI_MISO: R3.1 U6.2(SO) ; also sheet 1
GP7_SPI_MOSI: R4.1 U6.5(SI) ; also sheet 1
GP8_SD_CLK: USD.5(CLK) ; also sheet 1
GP9_SD_CMD: RP6.7 USD.3(CMD/DI) ; also sheet 1
GP10_SD_DAT0: RP6.5 USD.7(DAT0/DO) ; also sheet 1
GP11_SD_DAT1: R46.1 USD.8(DAT1) ; also sheet 1
GP12_SD_DAT2: RP6.1 USD.1(DAT2) ; also sheet 1
GP13_SD_DAT3: RP6.3 USD.2(DAT3/XCS) ; also sheet 1
N$6: R3.2 RE.C
N$7: LE.C R4.2
N$10: USD.11(CD2)
N$17: PWR.C R64.2
N$19: USD.12(CD1)
N$21: R65.1 U11.4(O)
N$22: C7.1 Q1.1(G) R65.2
N$23: C60.1 Q1.3(D) R67.1 USD.4(VDD)
N$24: R67.2 SDPW.A
N$55: JP1.2 R63.2
N$114: R55.1 X1.4(ID)
N$167: BUT1.P1 BUT1.P2 R56.1
N$168: BUT2.P1 BUT2.P2 R58.1
RX_RV: R53.1 UART_RV.P$2 ; also sheet 1
RX_VSDSP: R34.1 UART_VSDSP.P$2 ; also sheet 1
TX_RV: R54.1 UART_RV.P$3 ; also sheet 1
TX_VSDSP: R33.1 UART_VSDSP.P$3 ; also sheet 1
USB_RV+: X1.3(DATA+) ; also sheet 1
USB_RV-: X1.2(DATA-) ; also sheet 1

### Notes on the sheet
- SPI flash
- USB mini
- buttons
- SD card
- regulators
- 3.3v
- 1.2v
- 1.8v
- UART pinheaders
- PWR led

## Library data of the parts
ADC_JACK HP-OUT = Samin_e7:CON_3M5_4WAY_JACK
BUT1 BUT2 RESET = 121_PanunKomponentit:SW_SMD-SW-4_5.1X5.1X2.5_TS-1187A-C-E-B
C1-C35 C37-C59 C61-C76 C100-C121 = resistor:C-EU: CAPACITOR, European symbol
C60 = rcl:C-EU: CAPACITOR, European symbol
FB1-FB6 = Samin_e7:BLM: Ferrite bead
J1 = Samin_e7:JXD7-0V0XNL: RJ45 PulseJack w/LEDs
JMP1 = Samin_e7:0R-JMP: SMD 0R 0603 Jumper
JP1 = pinhead:PINHD-1X2: PIN HEADER
JP2 = pinhead:PINHD-1X3: PIN HEADER
JP3 = pinhead:PINHD-1X4: PIN HEADER
LE PWR RE SDPW = 121_PanunKomponentit:LED_0603
Q1 = Antimode_X1_X2:DMP3098L
R1-R17 R19-R37 R40 R41 R43-R46 R48-R67 R100 = rcl:R-US_: RESISTOR, American symbol
R18 = Antimode_X1_X2:R-US_: RESISTOR, American symbol
RP1-RP6 = Antimode_X1_X2:RESPAK-4X1206
TP1 TP_D1-TP_D16 TP_DQSC1 TP_DQSC2 TP_DQST1 TP_DQST2 = testpad:TP: Test pad
TV1 TV2 = Antimode_X1_X2:CG0603MLA-5.5ME: Transient voltage suppressor
U1 = 121_PanunKomponentit:VSRVES01
U2 = 121_PanunKomponentit:KSZ9131RNX
U3 = Samin_e7:TLV172
U4 = 121_PanunKomponentit:TPA6139A2
U5 U7 = Antimode_X1_X2:TLV2172IDGKR_8VSSOP
U6 = 121_PanunKomponentit:SPI_FLASH_WIDE_AND_NARROW
U8-U10 = audio_modules:ZXCL280E5TA
U11 = 74xx-little-de:74*1G08: 2-input AND gate
U100 = Samin_e7:IS43LD16640C-25BLI; BUILT_BY: EMA_Cory; COPYRIGHT: Copyright (C) 2018 Accelerated Designs. All rights reserved; DATASHEET: http://www.issi.com/WW/pdf/43-46LD16640C-32320C.pdf; MANUFACTURER_PART_NUMBER: IS43LD16640C-25BLI; SOURCELIBRARY: ISSI_2020-08-11; VENDOR: ISSI
UART_RV UART_VSDSP = 121_PanunKomponentit:4X1_2.54MM_CON
USD = Samin_e7:CON-USD: Micro SD connector
X1 = 121_PanunKomponentit:USB_MINI_KOREAN_U-M-M5SS-W-2_C91144
XC1 XC2 = audio_modules:CPOL-EU: POLARIZED CAPACITOR, European symbol
XTAL1 = 121_PanunKomponentit:CRYSTAL_3.2X2.5_NEW
XTAL2 = Antimode_X1_X2:CRYSTAL: CRYSTAL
